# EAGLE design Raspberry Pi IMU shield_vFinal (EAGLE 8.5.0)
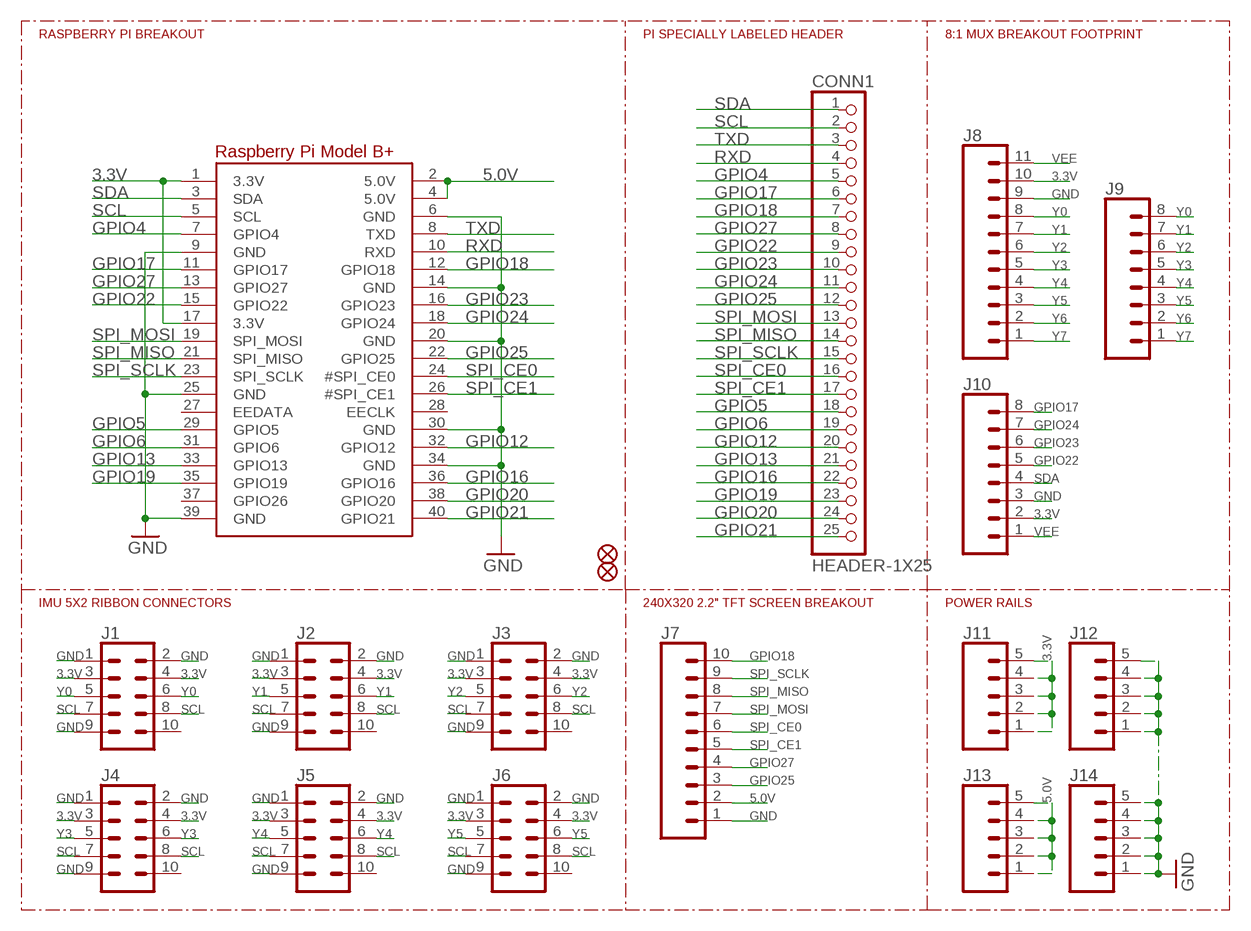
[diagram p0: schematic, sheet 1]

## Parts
CONN1  HEADER-1X25  [1X25_ROUND_70MIL]
FID2  FIDUCIAL""  [FIDUCIAL_1MM]
FID3  FIDUCIAL""  [FIDUCIAL_1MM]
J1  CONN_05X2SHD  [2X5-SHROUDED]
J2  CONN_05X2SHD  [2X5-SHROUDED]
J3  CONN_05X2SHD  [2X5-SHROUDED]
J4  CONN_05X2SHD  [2X5-SHROUDED]
J5  CONN_05X2SHD  [2X5-SHROUDED]
J6  CONN_05X2SHD  [2X5-SHROUDED]
J7  CONN_10LOCK  [1X10_LOCK]
J8  CONN_111X11_NO_SILK_KIT  [1X11_NO_SILK_KIT]
J9  CONN_08NO_SILK_FEMALE_PTH  [1X08_NO_SILK]
J10  CONN_08NO_SILK_FEMALE_PTH  [1X08_NO_SILK]
J11  CONN_05  [1X05]
J12  CONN_05  [1X05]
J13  CONN_05  [1X05]
J14  CONN_05  [1X05]
RPI1  RASPBERRYPI_BPLUS_HATNOSLOTS  [PI_HAT_NOSLOTS]

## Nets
3.3V [power]: J1.3 J1.4 J2.3 J2.4 J3.3 J3.4 J4.3 J4.4 J5.3 J5.4 J6.3 J6.4 J8.10 J10.2 J11.1 J11.2 J11.3 J11.4 J11.5 RPI1.1(3.3V) RPI1.17(3.3V)
5.0V [power]: J7.2 J13.1 J13.2 J13.3 J13.4 J13.5 RPI1.2(5.0V) RPI1.4(5.0V)
GND [power]: J1.1 J1.2 J1.9 J2.1 J2.2 J2.9 J3.1 J3.2 J3.9 J4.1 J4.2 J4.9 J5.1 J5.2 J5.9 J6.1 J6.2 J6.9 J7.1 J8.9 J10.3 J12.1 J12.2 J12.3 J12.4 J12.5 J14.1 J14.2 J14.3 J14.4 J14.5 RPI1.6(GND) RPI1.9(GND) RPI1.14(GND) RPI1.20(GND) RPI1.25(GND) RPI1.30(GND) RPI1.34(GND) RPI1.39(GND)
GPIO4: CONN1.5 RPI1.7(GPIO4)
GPIO5: CONN1.18 RPI1.29(GPIO5)
GPIO6: CONN1.19 RPI1.31(GPIO6)
GPIO12: CONN1.20 RPI1.32(GPIO12)
GPIO13: CONN1.21 RPI1.33(GPIO13)
GPIO16: CONN1.22 RPI1.36(GPIO16)
GPIO17: CONN1.6 J10.8 RPI1.11(GPIO17)
GPIO18: CONN1.7 J7.10 RPI1.12(GPIO18)
GPIO19: CONN1.23 RPI1.35(GPIO19)
GPIO20: CONN1.24 RPI1.38(GPIO20)
GPIO21: CONN1.25 RPI1.40(GPIO21)
GPIO22: CONN1.9 J10.5 RPI1.15(GPIO22)
GPIO23: CONN1.10 J10.6 RPI1.16(GPIO23)
GPIO24: CONN1.11 J10.7 RPI1.18(GPIO24)
GPIO25: CONN1.12 J7.3 RPI1.22(GPIO25)
GPIO27: CONN1.8 J7.4 RPI1.13(GPIO27)
RXD: CONN1.4 RPI1.10(RXD)
SCL: CONN1.2 J1.7 J1.8 J2.7 J2.8 J3.7 J3.8 J4.7 J4.8 J5.7 J5.8 J6.7 J6.8 RPI1.5(SCL)
SDA: CONN1.1 J10.4 RPI1.3(SDA)
SPI_CE0: CONN1.16 J7.6 RPI1.24(#SPI_CE0)
SPI_CE1: CONN1.17 J7.5 RPI1.26(#SPI_CE1)
SPI_MISO: CONN1.14 J7.8 RPI1.21(SPI_MISO)
SPI_MOSI: CONN1.13 J7.7 RPI1.19(SPI_MOSI)
SPI_SCLK: CONN1.15 J7.9 RPI1.23(SPI_SCLK)
TXD: CONN1.3 RPI1.8(TXD)
VEE [power]: J8.11 J10.1
Y0 [power]: J1.5 J1.6 J8.8 J9.8
Y1 [power]: J2.5 J2.6 J8.7 J9.7
Y2 [power]: J3.5 J3.6 J8.6 J9.6
Y3 [power]: J4.5 J4.6 J8.5 J9.5
Y4 [power]: J5.5 J5.6 J8.4 J9.4
Y5 [power]: J6.5 J6.6 J8.3 J9.3
Y6 [power]: J8.2 J9.2
Y7 [power]: J8.1 J9.1
Unconnected: J1.10 J2.10 J3.10 J4.10 J5.10 J6.10 RPI1.27(EEDATA) RPI1.28(EECLK) RPI1.37(GPIO26)

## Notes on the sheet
- RASPBERRY PI BREAKOUT | PI SPECIALLY LABELED HEADER | 8:1 MUX BREAKOUT FOOTPRINT
- IMU 5X2 RIBBON CONNECTORS | 240X320 2.2" TFT SCREEN BREAKOUT | POWER RAILS

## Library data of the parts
CONN1 = microbuilder:HEADER-1X25
FID2 FID3 = microbuilder:FIDUCIAL: Fiducial Alignment Points; BOM: EXCLUDE
J1-J6 = SparkFun-Connectors:CONN_05X2: Multi connection point. Often used as Generic Header-pin footprint for 0.1 inch spaced/style header connections For AVR SPI programming port, see special device with nice symbol: "AVR_SPI_PROG_5x2.dev" You can populate with any combo of single row headers, but if you'd like an exact match, check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; PROD_ID: CONN-08671; SF_ID: PRT-08506
J7 = SparkFun-Connectors:CONN_10: Multi connection point. Often used as Generic Header-pin footprint for 0.1 inch spaced/style header connections On any of the 0.1 inch spaced packages, you can populate with these: Break Away Headers - Straight (PRT-00116) Break Away Male Headers - Right Angle (PRT-00553) Female Headers (PRT-00115)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
J8 = SparkFun-Connectors:CONN_11: Multi connection point. Often used as Generic Header-pin footprint for 0.1 inch spaced/style header connections On any of the 0.1 inch spaced packages, you can populate with these: Break Away Headers - Straight (PRT-00116) Break Away Male Headers - Right Angle (PRT-00553) Female Headers (PRT-00115)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
J9 J10 = SparkFun-Connectors:CONN_08: Multi connection point. Often used as Generic Header-pin footprint for 0.1 inch spaced/style header connections On any of the 0.1 inch spaced packages, you can populate with these: Break Away Headers - Straight (PRT-00116) Break Away Male Headers - Right Angle (PRT-00553) Female Headers (PRT-00115)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; PROD_ID: CONN-08438
J11-J14 = SparkFun-Connectors:CONN_05: Multi connection point. Often used as Generic Header-pin footprint for 0.1 inch spaced/style header connections On any of the 0.1 inch spaced packages, you can populate with these: Break Away Headers - Straight (PRT-00116) Break Away Male Headers - Right Angle (PRT-00553) Female Headers (PRT-00115)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
RPI1 = microbuilder:RASPBERRYPI_BPLUS

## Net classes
0 default: width 0.254 mm, clearance 0.203 mm
1 power: width 0.406 mm, clearance 0.203 mm

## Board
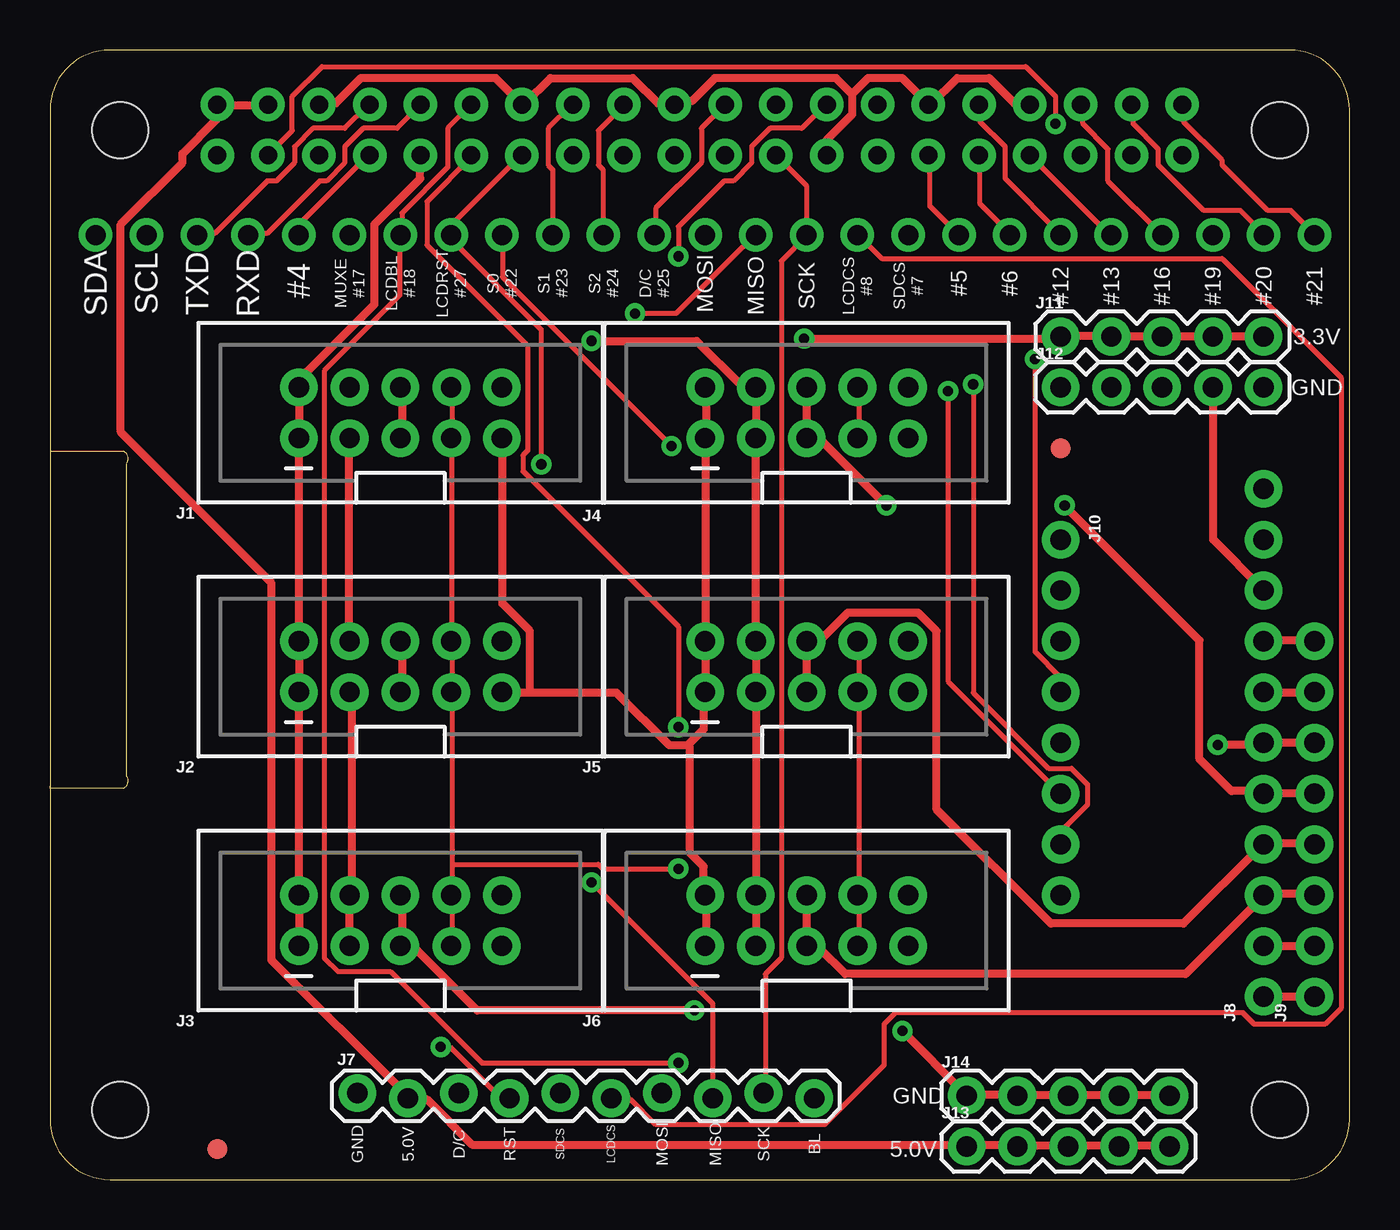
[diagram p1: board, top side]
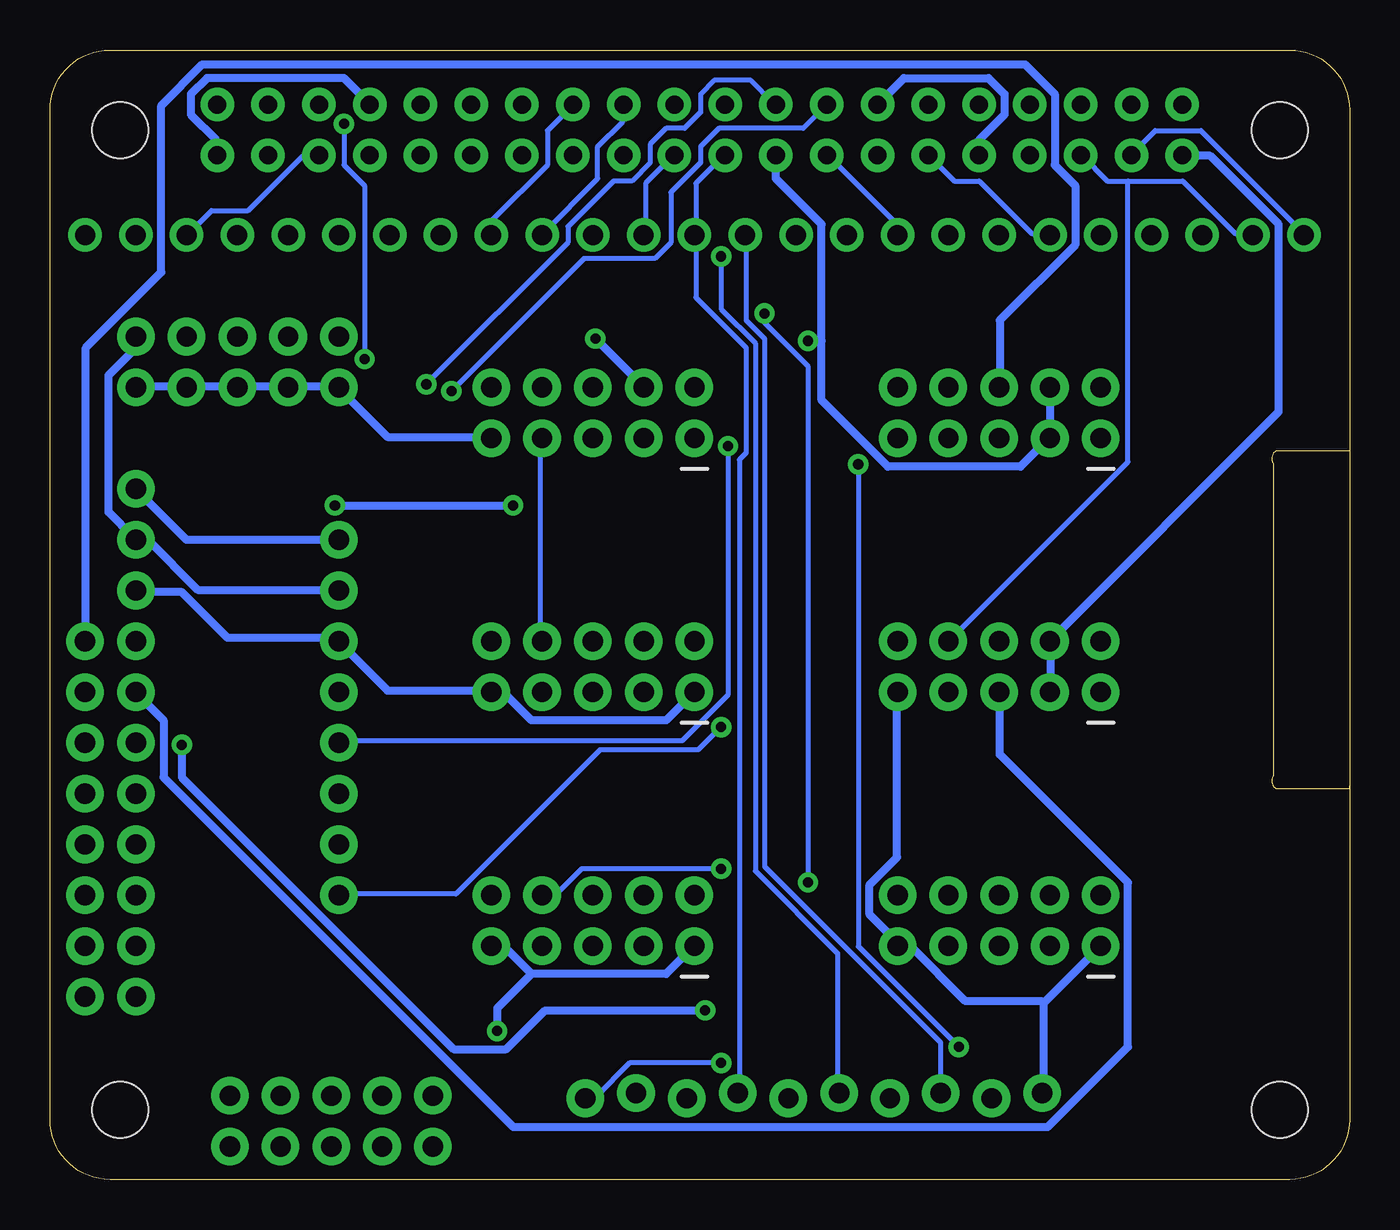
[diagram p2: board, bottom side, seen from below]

Size 65 x 56.5 mm. Coordinates in mm from the lower left corner, seen from the top.
Outline: 0,36.45 3.68,36.45 arc-90 3.81,35.81 3.81,20.19 arc-90 3.68,19.56 0,19.56 0,19.68
Copper layers (1*16): Top 0.035mm / dielectric 1.5mm / Bottom 0.035mm
Design rules "SparkFun": minimum track width 8mil, minimum drill 20mil, track to track 8mil, track to pad 8mil, pad to pad 8mil, via to via 8mil, smd to smd 8mil, copper to edge 10mil, drill to drill 8mil, minimum pad ring 12mil, minimum via ring 10mil, stop-mask expansion 4mil, vias tented up to drill 25mil, thermal gap 10mil

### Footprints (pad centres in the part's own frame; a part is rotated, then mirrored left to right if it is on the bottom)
1X25_ROUND_70MIL = drill 1 pad 1.676: 1 -30.48,0; 2 -27.94,0; 3 -25.4,0; 4 -22.86,0; 5 -20.32,0; 6 -17.78,0; 7 -15.24,0; 8 -12.7,0; 9 -10.16,0; 10 -7.62,0; 11 -5.08,0; 12 -2.54,0; 13 0,0; 14 2.54,0; 15 5.08,0; 16 7.62,0; 17 10.16,0; 18 12.7,0; 19 15.24,0; 20 17.78,0; 21 20.32,0; 22 22.86,0; 23 25.4,0; 24 27.94,0; 25 30.48,0
FIDUCIAL_1MM = smd 1 x 1: 1 0,0
2X5-SHROUDED = drill 1.016 pad 1.88: 1 -1.27,5.08; 2 1.27,5.08; 3 -1.27,2.54; 4 1.27,2.54; 5 -1.27,0; 6 1.27,0; 7 -1.27,-2.54; 8 1.27,-2.54; 9 -1.27,-5.08; 10 1.27,-5.08
1X10_LOCK = drill 1.016 pad 1.88: 1 0,0.127; 2 2.54,-0.127; 3 5.08,0.127; 4 7.62,-0.127; 5 10.16,0.127; 6 12.7,-0.127; 7 15.24,0.127; 8 17.78,-0.127; 9 20.32,0.127; 10 22.86,-0.127
1X11_NO_SILK_KIT = drill 1.016 pad 1.88: 1 0,0; 2 2.54,0; 3 5.08,0; 4 7.62,0; 5 10.16,0; 6 12.7,0; 7 15.24,0; 8 17.78,0; 9 20.32,0; 10 22.86,0; 11 25.4,0
1X08_NO_SILK = drill 1.016 pad 1.88: 1 0,0; 2 2.54,0; 3 5.08,0; 4 7.62,0; 5 10.16,0; 6 12.7,0; 7 15.24,0; 8 17.78,0
1X05 = drill 1.016 pad 1.88: 1 0,0; 2 2.54,0; 3 5.08,0; 4 7.62,0; 5 10.16,0
PI_HAT_NOSLOTS = drill 0.9 pad 1.676: 1 8.37,51.23; 2 8.37,53.77; 3 10.91,51.23; 4 10.91,53.77; 5 13.45,51.23; 6 13.45,53.77; 7 15.99,51.23; 8 15.99,53.77; 9 18.53,51.23; 10 18.53,53.77; 11 21.07,51.23; 12 21.07,53.77; 13 23.61,51.23; 14 23.61,53.77; 15 26.15,51.23; 16 26.15,53.77; 17 28.69,51.23; 18 28.69,53.77; 19 31.23,51.23; 20 31.23,53.77; 21 33.77,51.23; 22 33.77,53.77; 23 36.31,51.23; 24 36.31,53.77; 25 38.85,51.23; 26 38.85,53.77; 27 41.39,51.23; 28 41.39,53.77; 29 43.93,51.23; 30 43.93,53.77; 31 46.47,51.23; 32 46.47,53.77; 33 49.01,51.23; 34 49.01,53.77; 35 51.55,51.23; 36 51.55,53.77; 37 54.09,51.23; 38 54.09,53.77; 39 56.63,51.23; 40 56.63,53.77 | hole 2.8: 3.5,3.5; 3.5,52.5; 61.5,52.5; 61.5,3.5

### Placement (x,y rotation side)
CONN1  32.77,47.24 0 top
FID2  8.38,1.52 0 top
FID3  50.55,36.58 0 top
J1  17.53,38.35 90 top
J2  17.53,25.65 90 top
J3  17.53,12.95 90 top
J4  37.85,38.35 90 top
J5  37.85,25.65 90 top
J6  37.85,12.95 90 top
J7  15.37,4.19 0 top
J8  60.71,9.14 90 top
J9  63.25,9.14 90 top
J10  50.55,32 270 top
J11  50.55,42.16 0 top
J12  50.55,39.62 0 top
J13  45.85,1.65 0 top
J14  45.85,4.19 0 top
RPI1  0,0 0 top

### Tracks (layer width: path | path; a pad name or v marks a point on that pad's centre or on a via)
3.3V  (via drill 0.51)
  Top 0.406: J11.5 60.69,42.18 58.29,42.18 J11.4 58.06,42.18 55.78,42.18 J11.3 55.55,42.18 53.26,42.18 J11.2 53.03,42.18 50.63,42.18 J11.1 50.41,42.06 v37.72,42.06 | J6.3 35.32,11.77 35.32,14.17 J6.4 35.32,14.4 35.32,24.23 J5.3 35.32,24.46 35.32,26.86 J5.4 35.32,27.09 35.32,36.92 J4.3 35.32,37.15 35.32,39.55 J4.4 35.2,39.78 34.52,39.78 32.35,41.95 v27.09,41.95 | J3.3 14.97,11.77 14.97,14.17 J3.4 15.09,14.4 15.09,24.35 J2.3 | J1.3 14.97,37.03 14.97,26.98 J2.4
  Bottom 0.406: J10.2 50.63,29.49 57.61,29.49 60.12,32 J8.10 60.81,32.12 62.06,33.38 62.06,40.23 60.81,41.49 60.81,42.06 J11.5 | v37.72,42.06 35.32,39.66 J4.4 | 26.4,41.95 26.4,38.98 23.09,35.66 16.46,35.66 15.09,37.03 J1.3 14.97,37.26 14.97,39.55 J1.4 | 26.4,41.95 26.4,47.78 28.69,50.06 28.69,51.21 RPI1.17 | RPI1.1 8.34,51.21 6.97,51.21 3.54,47.78 3.54,38.41 14.97,26.98 J2.4 14.97,26.75 14.97,24.46 J2.3 | 26.4,41.95 v27.09,41.95
5.0V
  Top 0.406: RPI1.4 10.86,53.72 8.46,53.72 RPI1.2 8.34,53.61 8.34,53.03 6.63,51.32 6.63,50.86 3.54,47.78 3.54,37.38 11.09,29.83 11.09,10.97 17.83,4.23 J7.2 17.95,4 18.86,4 21.14,1.71 45.72,1.71 J13.1 45.95,1.71 48.35,1.71 J13.2 48.58,1.71 50.86,1.71 J13.3 51.09,1.71 53.38,1.71 J13.4 53.61,1.71 56.01,1.71 J13.5
GND  (via drill 0.51)
  Top 0.406: J12.4 58.18,39.55 58.18,32 60.69,29.49 J8.9 | J4.2 32.8,39.55 32.8,37.15 J4.1 32.8,36.92 32.8,27.09 J5.2 32.8,26.86 32.8,24.57 J5.1 32.69,24.35 32.69,22.52 31.89,21.72 | 24,24.35 28.35,24.35 30.98,21.72 31.89,21.72 | 24,24.35 22.63,24.35 J2.9 | 24,24.35 24,27.43 22.63,28.8 22.63,37.03 J1.9 | J14.5 56.01,4.23 53.61,4.23 J14.4 53.38,4.23 51.09,4.23 J14.3 50.86,4.23 48.58,4.23 J14.2 48.35,4.23 45.95,4.23 J14.1 45.72,4.34 v42.63,7.43 | J6.1 32.8,11.77 32.8,14.17 J6.2 32.69,14.4 32.69,15.66 32,16.34 32,21.6 31.89,21.72 | RPI1.6 13.49,53.84 14.29,53.84 15.54,55.09 22.29,55.09 23.55,53.84 RPI1.14 23.77,53.84 25.03,55.09 29.15,55.09 30.4,53.84 31.2,53.84 RPI1.20 31.32,53.95 32.12,53.95 33.26,55.09 39.32,55.09 40.12,54.29 | 40.12,54.29 40.12,53.26 38.86,52.01 38.86,51.32 RPI1.25 | 40.12,54.29 40.92,55.09 42.63,55.09 43.89,53.84 RPI1.30 44.12,53.84 45.38,55.09 46.98,55.09 48.23,53.84 48.92,53.84 RPI1.34 | J3.1 12.46,11.77 12.46,14.17 J3.2 12.46,14.4 12.46,24.23 J2.1 12.46,24.46 12.46,26.86 J2.2 12.46,27.09 12.46,36.92 J1.1 12.46,37.15 12.46,39.55 J1.2 12.57,39.78 12.57,40.12 16.23,43.78 16.23,47.78 18.52,50.06 18.52,51.21 RPI1.9
  Bottom 0.406: J4.9 42.98,37.15 48.12,37.15 50.52,39.55 J12.1 50.75,39.66 53.03,39.66 J12.2 53.26,39.66 55.55,39.66 J12.3 55.78,39.66 58.06,39.66 J12.4 58.29,39.66 60.69,39.66 J12.5 | J8.9 60.69,29.38 58.41,29.38 56.12,27.09 50.63,27.09 J10.3 50.52,26.86 48.12,24.46 42.98,24.46 J5.9 42.75,24.35 42.29,24.35 40.92,22.97 34.18,22.97 J5.1 | 40.92,10.29 42.29,11.66 42.86,11.66 J6.9 | 40.92,10.29 34.18,10.29 32.8,11.66 J6.1 | v42.63,7.43 42.63,8.57 40.92,10.29 | RPI1.9 18.52,51.32 18.52,52.01 17.26,53.26 17.26,54.29 18.06,55.09 22.29,55.09 23.55,53.84 RPI1.14 | RPI1.39 56.69,51.32 56.69,52.01 57.95,53.26 57.95,54.29 57.15,55.09 50.29,55.09 49.03,53.84 RPI1.34 | 15.32,8.8 15.32,4.34 J7.1 | 15.32,8.8 12.46,11.66 J3.1 | 15.32,8.8 15.43,8.91 19.2,8.91 21.95,11.66 22.52,11.66 J3.9 22.63,11.89 24,13.26 24,14.74 22.63,16.12 22.63,24.35 J2.9
GPIO4
  Top 0.254: CONN1.5 12.46,47.32 12.46,47.78 15.89,51.21 RPI1.7
GPIO5
  Top 0.254: RPI1.29 44.01,51.21 44.01,48.69 45.38,47.32 CONN1.18
GPIO6
  Top 0.254: RPI1.31 46.52,51.21 46.52,48.81 48.01,47.32 CONN1.19
GPIO12
  Top 0.254: RPI1.32 46.52,53.72 46.52,52.92 47.78,51.66 47.78,50.06 50.52,47.32 CONN1.20
GPIO13
  Top 0.254: RPI1.33 49.03,51.21 53.03,47.21 CONN1.21
GPIO16
  Top 0.254: CONN1.22 52.92,49.95 52.92,51.55 51.66,52.81 51.66,53.72 RPI1.36
GPIO17  (via drill 0.51)
  Top 0.254: v31.43,22.63 31.43,27.66 23.66,35.43 23.66,36.23 23.89,36.46 23.89,41.72 18.86,46.75 18.86,48.92 21.14,51.21 RPI1.11
  Bottom 0.254: CONN1.6 15.09,47.32 15.89,47.32 18.52,49.95 19.77,49.95 21.03,51.21 RPI1.11 | v31.43,22.63 32.58,21.49 37.49,21.49 44.69,14.29 50.52,14.29 J10.8
GPIO18  (via drill 0.51)
  Top 0.254: RPI1.12 21.03,53.72 19.89,52.58 19.89,50.63 17.6,48.35 17.6,47.32 CONN1.7 17.49,47.21 17.49,44.23 13.72,40.46 13.72,11.09 14.4,10.4 17.03,10.4 21.6,5.83 v31.43,5.83
  Bottom 0.254: v31.43,5.83 36.01,5.83 37.72,4.12 38.18,4.12 J7.10
GPIO19
  Bottom 0.254: RPI1.35 51.66,51.21 52.35,51.21 55.09,48.46 56.92,48.46 58.06,47.32 CONN1.23
GPIO20
  Top 0.254: RPI1.38 54.18,53.72 54.18,52.81 55.44,51.55 55.44,50.75 57.72,48.46 59.55,48.46 60.69,47.32 CONN1.24
GPIO21
  Top 0.254: RPI1.40 56.69,53.72 56.69,52.92 58.64,50.98 58.64,50.75 60.92,48.46 62.06,48.46 63.21,47.32 CONN1.25
GPIO22  (via drill 0.51)
  Top 0.254: v31.09,36.69 22.63,45.15 22.63,47.21 CONN1.9
  Bottom 0.254: CONN1.9 22.63,47.32 22.63,47.78 26.06,51.21 RPI1.15 | v31.09,36.69 31.09,24.23 33.38,21.95 50.52,21.95 J10.5
GPIO23  (via drill 0.51)
  Top 0.254: CONN1.10 25.15,50.52 24.92,50.75 24.92,52.58 26.06,53.72 RPI1.16 | v44.92,39.43 44.92,24.92 50.52,19.32 J10.6
  Bottom 0.254: v44.92,39.43 38.29,46.06 34.75,46.06 33.95,46.86 33.95,49.38 32.46,50.86 32.46,51.66 31.55,52.58 27.32,52.58 26.18,53.72 RPI1.16
GPIO24  (via drill 0.51)
  Top 0.254: CONN1.11 27.66,47.32 27.66,50.52 27.43,50.75 27.43,52.46 28.69,53.72 RPI1.18 | v46.18,39.78 46.18,24.35 49.95,20.57 51.09,20.57 51.89,19.77 51.89,18.75 50.63,17.49 50.63,16.8 J10.7
  Bottom 0.254: v46.18,39.78 39.09,46.86 39.09,47.66 36.8,49.95 35.89,49.95 34.98,50.86 34.98,51.78 34.18,52.58 33.26,52.58 32.46,53.38 32.46,54.29 31.77,54.98 29.95,54.98 28.8,53.84 RPI1.18
GPIO25
  Top 0.254: CONN1.12 30.29,47.32 30.29,48.58 32.58,50.86 32.58,52.58 33.72,53.72 RPI1.22
  Bottom 0.254: J7.3 20.46,4.34 20.46,6.86 29.26,15.66 29.26,42.06 30.18,42.98 30.18,47.21 CONN1.12
GPIO27  (via drill 0.51)
  Top 0.254: RPI1.13 23.55,51.21 20.12,47.78 20.12,47.32 CONN1.8 20.12,47.21 20.12,46.98 24.57,42.52 v24.57,35.78 | v19.55,6.63 20,6.63 22.52,4.12 22.97,4.12 J7.4
  Bottom 0.254: v19.55,6.63 24.57,11.66 v24.57,35.78
RXD
  Top 0.254: CONN1.4 9.94,47.32 10.86,47.32 13.49,49.95 13.83,49.95 14.74,50.86 14.74,51.66 15.66,52.58 17.37,52.58 18.52,53.72 RPI1.10
SCL  (via drill 0.51)
  Top 0.254: J4.7 40.46,37.15 40.46,39.55 J4.8 | J6.7 40.46,11.77 40.46,14.17 J6.8 40.46,14.29 40.46,24.35 J5.7 40.46,24.46 40.46,26.86 J5.8 | J1.8 20.12,39.55 20.12,37.15 J1.7 20.12,37.03 20.12,26.98 J2.8 20.12,26.86 20.12,24.46 J2.7 20.12,24.35 20.12,15.77 | J3.7 20.12,11.77 20.12,14.17 J3.8 20.12,14.29 20.12,15.77 | v31.43,15.54 27.66,15.54 27.43,15.77 20.12,15.77
  Bottom 0.254: J4.7 40.46,37.03 40.46,26.98 J5.8 | 11.09,49.95 12.12,49.95 13.37,51.21 RPI1.5 | 11.09,49.95 8.34,49.95 5.71,47.32 4.92,47.32 CONN1.2 | 11.09,49.95 11.09,35.89 20,26.98 J2.8 | v31.43,15.54 38.41,15.54 39.66,14.29 40.35,14.29 J6.8
SDA  (via drill 0.51)
  Top 0.254: v49.26,41.03 49.26,26.4 50.52,25.15 50.52,24.46 J10.4 | v50.29,52.81 50.29,54.18 48.81,55.66 13.6,55.66 12.12,54.18 12.12,52.46 10.97,51.32 RPI1.3
  Bottom 0.254: CONN1.1 2.29,47.32 7.43,52.46 9.72,52.46 10.86,51.32 RPI1.3 | v49.26,41.03 49.26,49.72 50.29,50.75 v50.29,52.81
SPI_CE0
  Top 0.254: J7.6 28.12,4 29.03,4 30.29,2.74 38.75,2.74 41.72,5.71 41.72,7.77 42.29,8.34 59.66,8.34 60.24,7.77 63.78,7.77 64.58,8.57 64.58,40.12 58.64,46.06 41.6,46.06 40.46,47.21 CONN1.16
  Bottom 0.254: RPI1.24 36.35,53.72 36.35,52.92 37.6,51.66 37.6,50.06 40.35,47.32 CONN1.16
SPI_CE1  (via drill 0.51)
  Top 0.254: v31.43,46.18 31.43,47.66 33.72,49.95 34.18,49.95 35.09,50.86 35.09,51.66 36.01,52.58 37.6,52.58 38.75,53.72 RPI1.26
  Bottom 0.254: CONN1.17 42.86,47.32 42.86,48.01 40.12,50.75 40.12,52.46 38.86,53.72 RPI1.26 | v31.43,46.18 31.43,43.55 29.72,41.83 29.72,15.43 25.6,11.32 25.6,4.34 J7.5
SPI_MISO  (via drill 0.51)
  Top 0.254: J7.8 33.15,8.8 v27.09,14.86 | v29.26,43.32 31.32,43.32 35.2,47.21 CONN1.14
  Bottom 0.254: CONN1.14 35.2,47.32 35.2,49.84 33.83,51.21 RPI1.21 | v27.09,14.86 27.09,40.69 29.26,42.86 v29.26,43.32
SPI_MOSI
  Bottom 0.254: RPI1.19 31.32,51.21 32.69,49.84 32.69,47.32 CONN1.13 32.69,47.21 32.69,44.12 30.18,41.6 30.18,36.35 30.52,36.01 30.52,4.34 J7.7
SPI_SCLK
  Top 0.254: RPI1.23 36.35,51.21 37.83,49.72 37.83,47.32 CONN1.15 37.83,47.21 36.58,45.95 36.58,11.09 35.78,10.29 35.78,4.34 J7.9
TXD
  Top 0.254: CONN1.3 7.43,47.32 8.23,47.32 10.86,49.95 11.32,49.95 12.23,50.86 12.23,51.66 13.14,52.58 14.74,52.58 15.89,53.72 RPI1.8
VEE
  Bottom 0.406: J10.1 58.18,32 60.69,34.52 J8.11
Y0
  Top 0.406: J1.5 17.6,37.15 17.6,39.55 J1.6 | J8.8 60.81,26.98 63.21,26.98 J9.8
  Bottom 0.406: J1.6 17.49,39.66 17.49,42.98 13.72,46.75 13.72,49.72 14.74,50.75 14.74,54.29 16.23,55.78 57.38,55.78 59.44,53.72 59.44,45.38 63.21,41.6 63.21,26.98 J9.8
Y1
  Top 0.406: J2.5 17.6,24.46 17.6,26.86 J2.6 | J8.7 60.81,24.35 63.21,24.35 J9.7
  Bottom 0.406: J2.5 17.49,24.35 17.49,21.26 11.09,14.86 11.09,6.63 15.09,2.63 41.83,2.63 59.32,20.12 59.32,22.97 60.69,24.35 J8.7
Y2  (via drill 0.51)
  Top 0.406: J3.6 17.6,14.17 17.6,11.77 J3.5 17.72,11.66 18.17,11.66 21.37,8.46 v32.23,8.46 | J9.6 63.21,21.83 60.81,21.83 J8.6 60.22,21.74 v58.41,21.74
  Bottom 0.406: v32.23,8.46 40.23,8.46 42.18,6.51 44.81,6.51 58.41,20.12 v58.41,21.74
Y3  (via drill 0.51)
  Top 0.406: J4.6 37.83,39.55 37.83,37.15 J4.5 37.95,36.92 38.63,36.92 v41.83,33.72 | J9.5 63.21,19.32 60.81,19.32 J8.5 60.58,19.43 59.09,19.43 57.49,21.03 57.49,26.98 v50.75,33.72
  Bottom 0.406: v50.75,33.72 v41.83,33.72
Y4
  Top 0.406: J5.5 37.83,24.46 37.83,26.86 J5.6 37.95,27.09 38.63,27.09 39.89,28.35 43.43,28.35 44.35,27.43 44.35,18.52 50.06,12.8 56.69,12.8 60.58,16.69 J8.4 60.81,16.8 63.21,16.8 J9.4
Y5
  Top 0.406: J6.6 37.83,14.17 37.83,11.77 J6.5 37.95,11.54 38.52,11.54 39.78,10.29 56.81,10.29 60.58,14.06 J8.3 60.81,14.29 63.21,14.29 J9.3
Y6
  Top 0.406: J8.2 60.81,11.66 63.21,11.66 J9.2
Y7
  Top 0.406: J9.1 J8.1

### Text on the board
tPlace: SDA | SCL | TXD | RXD | #4 | MUXE / #17 | LCDBL / #18 | LCDRST / #27 | S0 / #22 | S1 / #23 | S2 / #24 | D/C / #25 | MOSI | MISO | SCK | LCDCS / #8 | SDCS / #7 | #5 | #6 | #12 | #13 | #16 | #19 | #20 | #21 | 3.3V | GND | GND | GND | 5.0V | D/C | RST | SDCS | LCDCS | MOSI | MISO | SCK | BL | 5.0V

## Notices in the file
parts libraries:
microbuilder: This work is placed in the public domain, and may be freely used for commercial and non-commercial work with the following conditions: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
SparkFun-Connectors: Licensing: Creative Commons ShareAlike 4.0 International - https://creativecommons.org/licenses/by-sa/4.0
